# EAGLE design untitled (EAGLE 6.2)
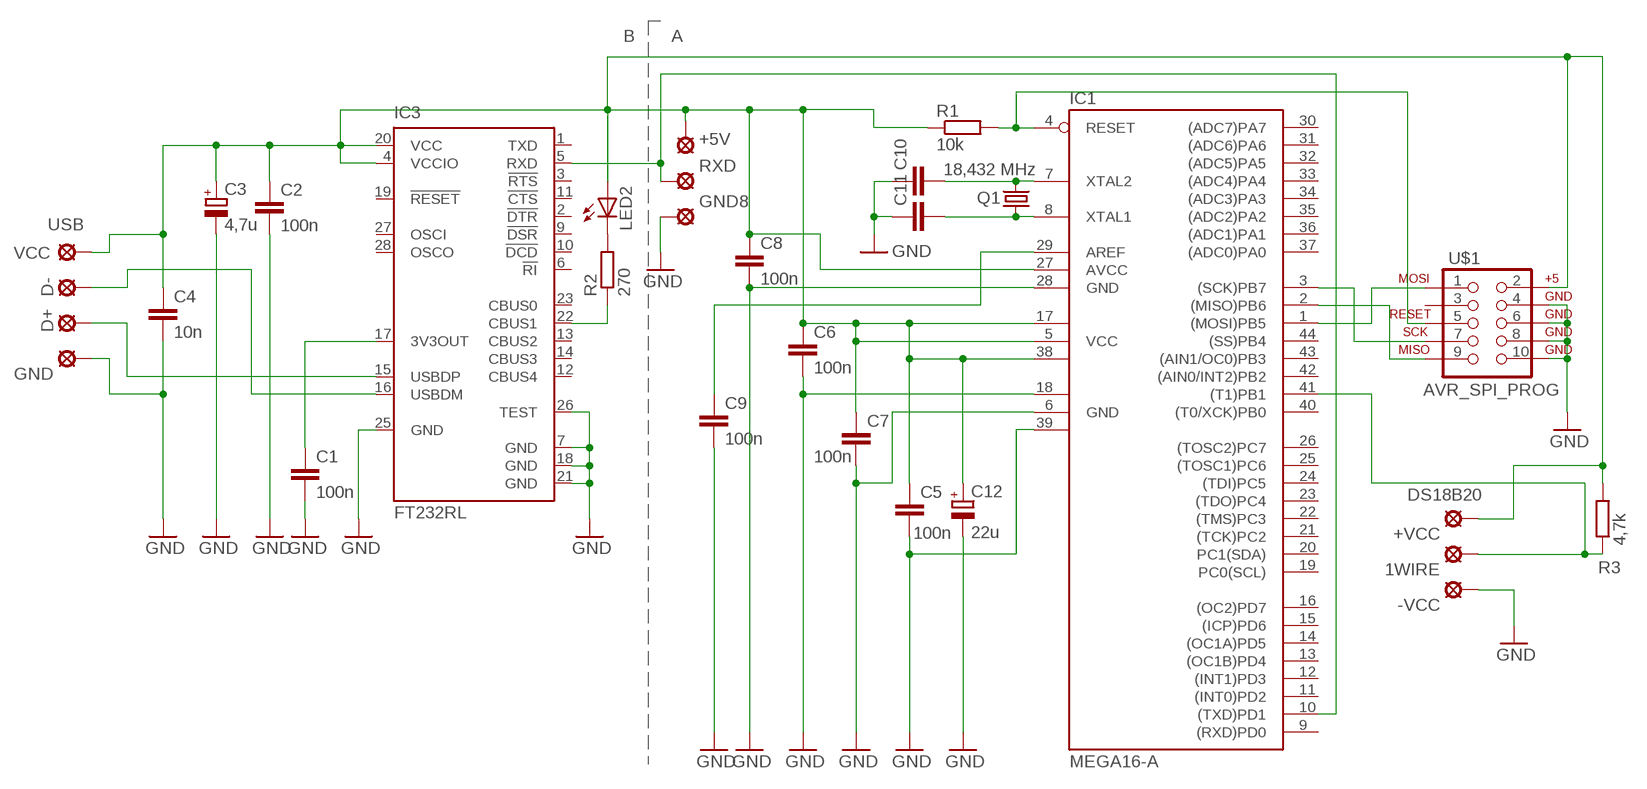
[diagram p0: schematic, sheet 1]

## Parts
1WIRE  LSP11  [LSP11]
+5V  LSP11  [LSP11]
+VCC  LSP11  [LSP11]
-VCC  LSP11  [LSP11]
C1  100n  C-EUC1210  [C1210]
C2  100n  C-EUC1210  [C1210]
C3  4,7u  CPOL-EU153CLV-0405  [153CLV-0405]
C4  10n  C-EUC1206  [C1206]
C5  100n  C-EUC1210  [C1210]
C6  100n  C-EUC1210  [C1210]
C7  100n  C-EUC1210  [C1210]
C8  100n  C-EUC1210  [C1210]
C9  100n  C-EUC1210  [C1210]
C10  C-EUC1206  [C1206]
C11  C-EUC1206  [C1206]
C12  22u  CPOL-EUUD-6,3X7,7  [UD-6,3X7,7_NICHICON]
D+  LSP11  [LSP11]
D-  LSP11  [LSP11]
GND  LSP11  [LSP11]
GND8  LSP11  [LSP11]
IC1  MEGA16-A  [TQFP44]
IC3  FT232RL  [SSOP28]
LED2  LED-FKIT-1206  [FKIT-LED-1206]
Q1  18,432 MHz  CRYSTALHC49S  [HC49/S]
R1  10k  R-EU_R1206  [R1206]
R2  270  R-EU_R1206  [R1206]
R3  4,7k  R-EU_R1206  [R1206]
RXD  LSP11  [LSP11]
U$1  AVR_SPI_PROG  [AVR_ICSP]
VCC  LSP11  [LSP11]

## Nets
GND: -VCC.MP C1.2 C2.2 C3.- C4.2 C5.2 C6.2 C7.2 C8.2 C9.2 C10.1 C11.1 C12.- GND8.MP GND.MP IC1.6(GND) IC1.18(GND1) IC1.28(GND) IC1.39(GND2) IC3.7(GND) IC3.18(GND) IC3.21(GND) IC3.25(GND) IC3.26(TEST) U$1.4 U$1.6 U$1.8 U$1.10
N$1: C1.1 IC3.17(3V3OUT)
N$2: D-.MP IC3.16(USBDM)
N$3: +5V.MP +VCC.MP C2.1 C3.+ C4.1 C5.1 C6.1 C7.1 C8.1 C12.+ IC1.5(VCC) IC1.17(VCC1) IC1.27(AVCC) IC1.38(VCC2) IC3.4(VCCIO) IC3.20(VCC) LED2.A R1.1 R3.2 U$1.2 VCC.MP
N$4: IC1.10((TXD)PD1) IC3.5(RXD) RXD.MP
N$5: IC1.1((MOSI)PB5) U$1.1
N$6: D+.MP IC3.15(USBDP)
N$7: IC1.3((SCK)PB7) U$1.7
N$8: IC3.22(CBUS1) R2.1
N$9: C10.2 IC1.7(XTAL2) Q1.2
N$10: LED2.C R2.2
N$11: C11.2 IC1.8(XTAL1) Q1.1
N$12: IC1.4(RESET) R1.2 U$1.5
N$13: IC1.2((MISO)PB6) U$1.9
N$14: C9.1 IC1.29(AREF)
N$16: 1WIRE.MP IC1.41((T1)PB1) R3.1
Unconnected: IC1.9((RXD)PD0) IC1.11((INT0)PD2) IC1.12((INT1)PD3) IC1.13((OC1B)PD4) IC1.14((OC1A)PD5) IC1.15((ICP)PD6) IC1.16((OC2)PD7) IC1.19(PC0(SCL)) IC1.20(PC1(SDA)) IC1.21((TCK)PC2) IC1.22((TMS)PC3) IC1.23((TDO)PC4) IC1.24((TDI)PC5) IC1.25((TOSC1)PC6) IC1.26((TOSC2)PC7) IC1.30((ADC7)PA7) IC1.31((ADC6)PA6) IC1.32((ADC5)PA5) IC1.33((ADC4)PA4) IC1.34((ADC3)PA3) IC1.35((ADC2)PA2) IC1.36((ADC1)PA1) IC1.37((ADC0)PA0) IC1.40((T0/XCK)PB0) IC1.42((AIN0/INT2)PB2) IC1.43((AIN1/OC0)PB3) IC1.44((SS)PB4) IC3.1(TXD) IC3.2(!DTR) IC3.3(!RTS) IC3.6(!RI) IC3.9(!DSR) IC3.10(!DCD) IC3.11(!CTS) IC3.12(CBUS4) IC3.13(CBUS2) IC3.14(CBUS3) IC3.19(!RESET) IC3.23(CBUS0) IC3.27(OSCI) IC3.28(OSCO) U$1.3

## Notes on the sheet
- B | A
- USB
- DS18B20

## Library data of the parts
1WIRE +5V +VCC -VCC D+ D- GND GND8 RXD VCC = solpad:LSP11: SOLDER PAD
C1 C2 C4-C11 = rcl:C-EU: CAPACITOR, European symbol
C3 C12 = rcl:CPOL-EU: POLARIZED CAPACITOR, European symbol
IC1 = atmel:MEGA16: MICROCONTROLLER 16 Kbytes FLASH 1 kbytes SRAM 512 bytes EEPROM USART 8-channel 10 bit ADC Source: avr.lbr; MPN: ATMEGA16-16AU; OC_FARNELL: 9171134; OC_NEWARK: 96K6515
IC3 = ftdichip:FT232R: Source: http://www.ftdichip.com/Documents/DataSheets/DS_FT232R_v104.pdf; MPN: FT232RL; OC_FARNELL: 1146032; OC_NEWARK: 91K9918
LED2 = SparkFun:LED: LEDs
Q1 = crystal:CRYSTAL: CRYSTAL; OC_FARNELL: 1667008; OC_NEWARK: unknown
R1-R3 = rcl:R-EU_: RESISTOR, European symbol
U$1 = SparkFun:AVR_SPI_PROG: AVR ICSP Header This is the standard AVR In Circuit Serial Programming header. Minimal, but includes pin one indicator. Works with standard Olimex programmers. Also look for the 6-pin reduced version. Spark Fun Electronics SKU: PRT-00778

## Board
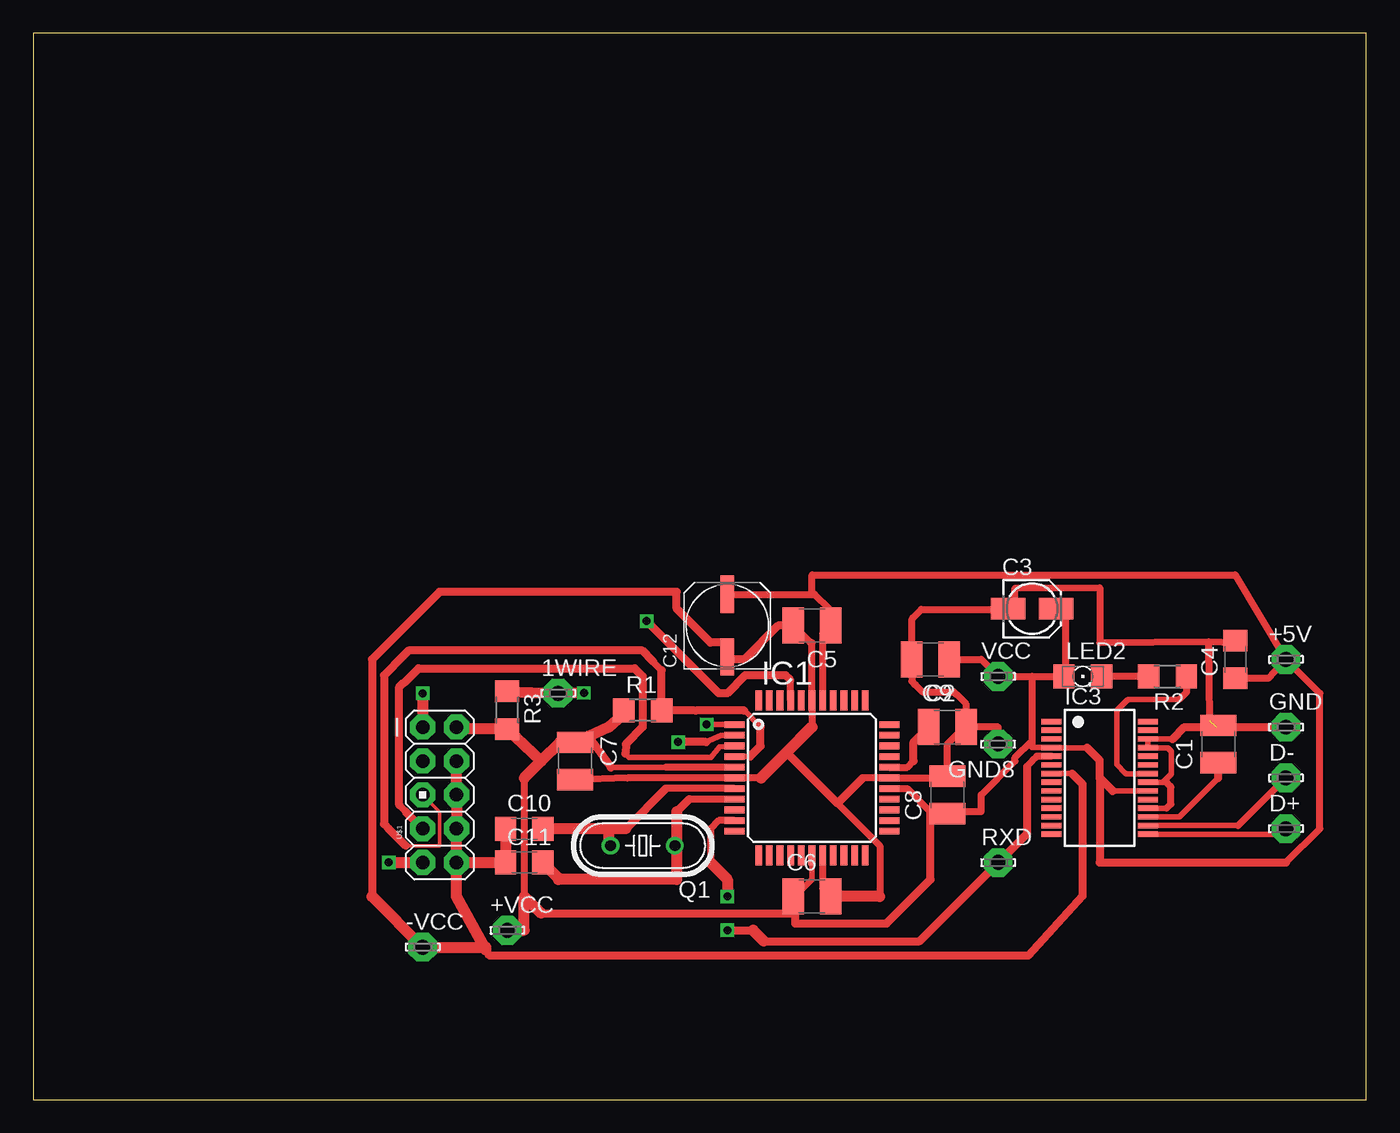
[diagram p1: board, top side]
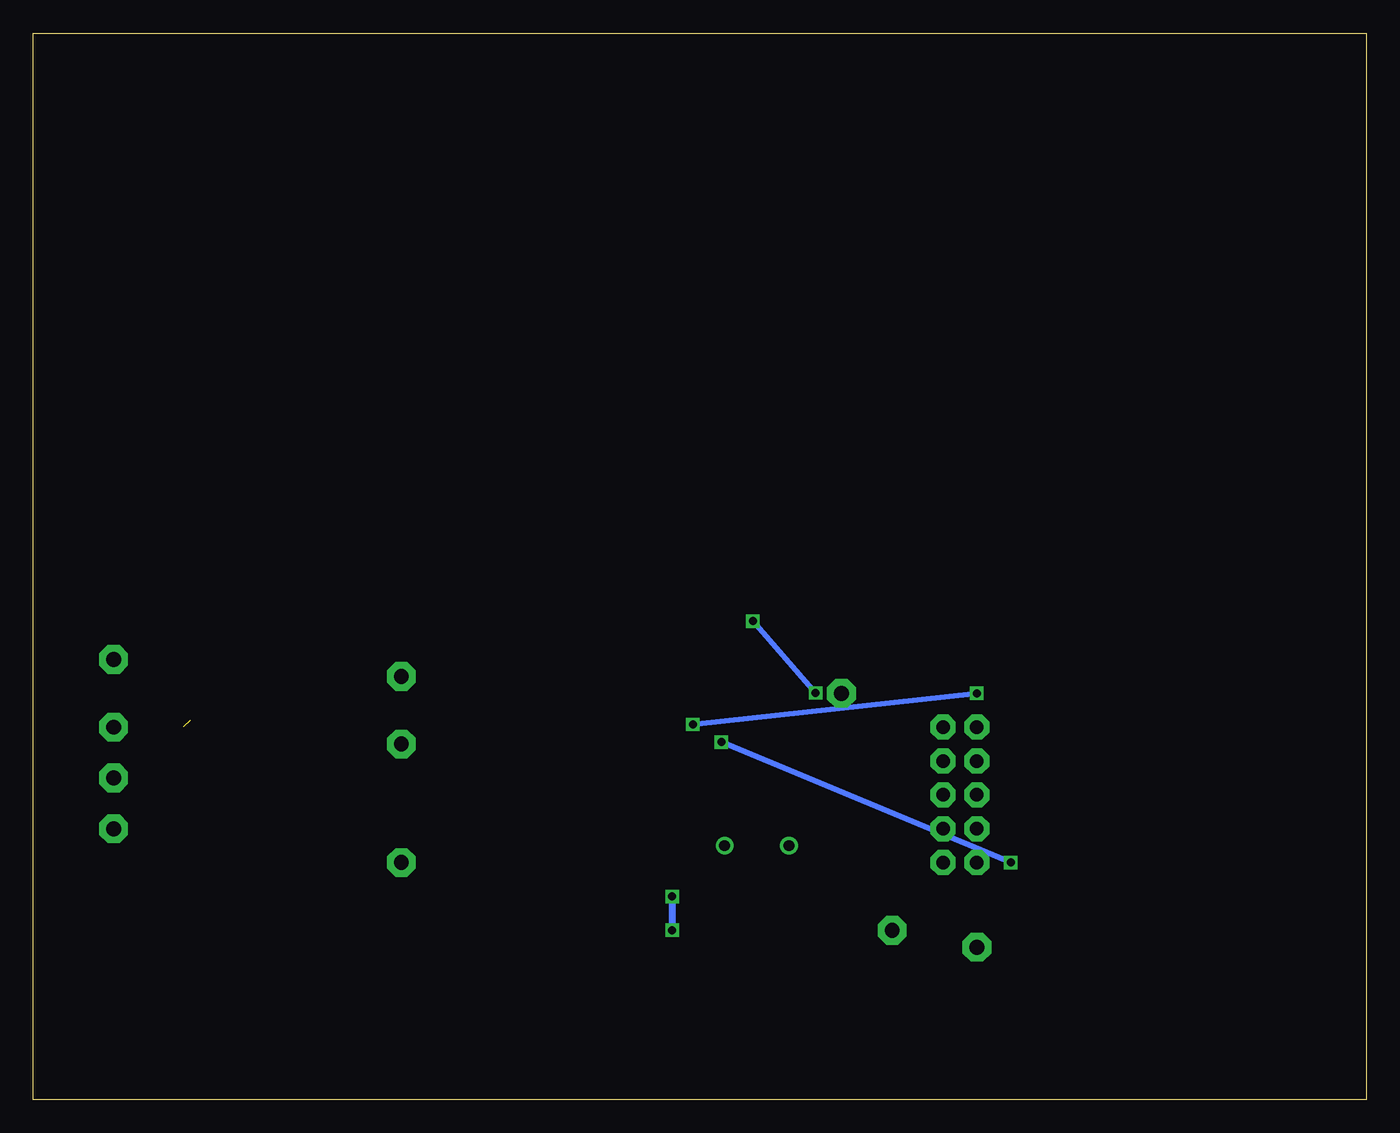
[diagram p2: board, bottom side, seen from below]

Size 100 x 80 mm. Coordinates in mm from the lower left corner, seen from the top.
Outline: 0,0 100,0 100,80 0,80 0,0
Copper layers (1*16): Top 0.035mm / dielectric 1.5mm / Bottom 0.035mm
Design rules: minimum track width 10mil, minimum drill 24mil, track to track 8mil, track to pad 8mil, pad to pad 8mil, via to via 8mil, smd to smd 8mil, copper to edge 40mil, drill to drill 8mil, minimum pad ring 10mil, minimum via ring 8mil, stop-mask expansion 4mil, vias tented up to drill 0mil, thermal gap 10mil

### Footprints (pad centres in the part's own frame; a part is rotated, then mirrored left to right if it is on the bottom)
LSP11 = drill 1.118 pad 2.159 octagon: MP 0,0
C1210 = smd 1.6 x 2.7: 1 -1.4,0; 2 1.4,0
153CLV-0405 = smd 2.6 x 1.6: + 1.8,0; - -1.8,0
C1206 = smd 1.6 x 1.8: 1 -1.4,0; 2 1.4,0
UD-6,3X7,7_NICHICON = smd 2.8 x 1: + 2.35,0; - -2.35,0
TQFP44 = smd 1.5 x 0.5: 1 -5.8,4; 2 -5.8,3.2; 3 -5.8,2.4; 4 -5.8,1.6; 5 -5.8,0.8; 6 -5.8,0; 7 -5.8,-0.8; 8 -5.8,-1.6; 9 -5.8,-2.4; 10 -5.8,-3.2; 11 -5.8,-4; 23 5.8,-4; 24 5.8,-3.2; 25 5.8,-2.4; 26 5.8,-1.6; 27 5.8,-0.8; 28 5.8,0; 29 5.8,0.8; 30 5.8,1.6; 31 5.8,2.4; 32 5.8,3.2; 33 5.8,4 | smd 0.5 x 1.5: 12 -4,-5.8; 13 -3.2,-5.8; 14 -2.4,-5.8; 15 -1.6,-5.8; 16 -0.8,-5.8; 17 0,-5.8; 18 0.8,-5.8; 19 1.6,-5.8; 20 2.4,-5.8; 21 3.2,-5.8; 22 4,-5.8; 34 4,5.8; 35 3.2,5.8; 36 2.4,5.8; 37 1.6,5.8; 38 0.8,5.8; 39 0,5.8; 40 -0.8,5.8; 41 -1.6,5.8; 42 -2.4,5.8; 43 -3.2,5.8; 44 -4,5.8
SSOP28 = smd 0.4 x 1.5: 1 -4.225,-3.625; 2 -3.575,-3.625; 3 -2.925,-3.625; 4 -2.275,-3.625; 5 -1.625,-3.625; 6 -0.975,-3.625; 7 -0.325,-3.625; 8 0.325,-3.625; 9 0.975,-3.625; 10 1.625,-3.625; 11 2.275,-3.625; 12 2.925,-3.625; 13 3.575,-3.625; 14 4.225,-3.625; 15 4.225,3.625; 16 3.575,3.625; 17 2.925,3.625; 18 2.275,3.625; 19 1.625,3.625; 20 0.975,3.625; 21 0.325,3.625; 22 -0.325,3.625; 23 -0.975,3.625; 24 -1.625,3.625; 25 -2.275,3.625; 26 -2.925,3.625; 27 -3.575,3.625; 28 -4.225,3.625
FKIT-LED-1206 = smd 1.6 x 1.803: A -1.422,0; C 1.422,0
HC49/S = drill 0.813: 1 -2.413,0; 2 2.413,0
R1206 = smd 1.6 x 1.803: 1 -1.422,0; 2 1.422,0
AVR_ICSP = drill 1.016 pad 1.88 octagon: 1 -1.27,5.08; 2 1.27,5.08; 3 -1.27,2.54; 4 1.27,2.54; 5 -1.27,0; 6 1.27,0; 7 -1.27,-2.54; 8 1.27,-2.54; 9 -1.27,-5.08; 10 1.27,-5.08

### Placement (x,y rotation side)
1WIRE  39.37,30.48 0 top
+5V  93.98,33.02 0 top
+VCC  35.56,12.7 0 top
-VCC  29.21,11.43 0 top
C1  88.9,26.67 90 top
C2  67.31,33.02 180 top
C3  74.93,36.83 0 top
C4  90.17,33.02 90 top
C5  58.42,35.56 180 top
C6  58.42,15.24 0 top
C7  40.64,25.4 270 top
C8  68.58,22.86 90 top
C9  68.58,27.94 0 top
C10  36.83,20.32 0 top
C11  36.83,17.78 0 top
C12  52.07,35.56 90 top
D+  93.98,20.32 0 top
D-  93.98,24.13 0 top
GND  93.98,27.94 0 top
GND8  72.39,26.67 180 top
IC1  58.42,24.13 0 top
IC3  80.01,24.13 270 top
LED2  78.74,31.75 0 top
Q1  45.72,19.05 180 top
R1  45.72,29.21 0 top
R2  85.09,31.75 180 top
R3  35.56,29.21 270 top
RXD  72.39,17.78 0 top
U$1  30.48,22.86 0 top
VCC  72.39,31.75 0 top

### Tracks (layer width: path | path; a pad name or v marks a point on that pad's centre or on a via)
GND  (1 unrouted)
  Top 0.254: 35.56,17.78 C11.1 | 35.56,20.32 C10.1 | 90.17,34.29 C4.2 | 67.31,36.83 C3.- 73.66,36.83 | 53.34,24.13 IC1.6 | 58.42,29.21 IC1.39 | 59.69,15.24 C6.2 | 63.5,24.13 IC1.28 | 69.85,27.94 C9.2 | 68.58,24.13 C8.2 | 52.07,34.29 C12.- | 88.9,27.94 C1.2
  Top 0.406: IC3.18 85.03,21.86 | 85.09,23.72 85.01,23.8 IC3.21 84.74,23.8 85.37,24.43 85.37,26.11 85.11,26.36 83.67,26.36 IC3.25 IC3.26 85.47,27.05 | 88.77,27.94 C1.2 | IC3.7 77.93,24.45 | 33.96,11.43 33.96,11.21
  Top 0.508: IC1.39 58.42,34.29 58.29,34.29 C5.2 | 52.26,33.02 C12.- | IC1.28 68.45,24.13 C8.2 68.58,26.67 69.85,27.94 | 88.16,34.37 90.17,34.29 | GND8.MP 72.39,27.94 C9.2 69.95,27.97 69.95,29.72 69.24,30.43 69.22,30.43 69.06,30.58 66.7,30.58 66.19,31.09 66.19,31.11 65.91,31.4 C2.2 65.91,36.01 65.99,36.09 65.99,36.14 66.62,36.78 73.08,36.78 C3.- | 63.5,15.24 63.5,19.05 60.33,22.23 | 88.16,34.37 80.01,34.29 80.01,38.41 73.66,38.38 73.66,36.83 | 85.03,21.86 85.34,22.17 85.34,23.44 85.32,23.47 85.32,23.5 85.09,23.72 | 63.5,24.13 62.23,24.13 | 58.42,29.21 58.42,27.94 58.4,27.94 | 54.61,24.13 53.34,24.13 | 56.49,26.04 56.52,26.04 | IC1.18 59.22,15.84 C6.2 | IC1.6 44.58,24.13 C7.2 | 88.16,34.37 88.24,28.45
  Top 0.61: C5.2 55.88,35.56 53.34,33.02 52.26,33.02 | 88.9,27.94 GND.MP | 85.47,27.05 86.36,27.94 88.77,27.94 | 62.23,24.13 60.33,22.23 56.52,26.04 | 77.93,24.45 78.72,23.67 78.72,15.27 74.62,10.79 34.24,10.79 33.96,11.21 | 52.07,34.29 50.8,34.29 48.26,36.83 48.26,38.1 30.48,38.1 25.4,33.02 25.4,15.24
  Top 0.813: C10.1 C11.1 U$1.10 | U$1.4 U$1.6 U$1.8 U$1.10 | 63.5,15.24 C6.2 | U$1.10 31.75,15.24 33.96,11.21 | 58.42,27.94 54.61,24.13 | 58.4,27.94 56.49,26.04 | 33.96,11.43 -VCC.MP 25.4,15.24
N$1
  Top 0.406: IC3.17 85.97,21.2 88.9,24.13
  Top 0.61: 88.9,24.13 C1.1
N$2
  Top 0.406: IC3.16 90.41,20.55
  Top 0.508: 90.41,20.55 D-.MP
N$3
  Top 0.254: 77.47,36.83 C3.+ | 77.47,31.75 LED2.A | 68.58,21.59 C8.1 67.31,21.59 | 57.15,15.24 C6.1
  Top 0.406: IC1.17 58.42,16.51 57.15,15.24 | IC3.20 80.98,23.16 | 79.07,26.39 IC3.4 74.93,26.41 74.93,26.67 | 47.46,24.93 43.33,24.92
  Top 0.508: IC1.38 59.23,29.93 59.23,34.97 C5.1 59.69,35.69 59.69,36.83 58.61,37.91 58.42,37.91 | C12.+ 58.42,37.91 | IC1.27 65.57,23.33 67.31,21.59 68.45,21.59 C8.1 | +5V.MP 90.17,39.37 58.42,39.37 58.42,37.91 | 74.93,31.75 VCC.MP 71.12,33.02 C2.1 | 74.93,31.75 LED2.A | 77.47,31.75 77.47,36.83 | 68.58,21.59 71.12,21.59 71.12,22.86 73.66,25.4 73.66,25.65 74.93,26.92 | 74.93,31.75 74.93,26.92 | 74.93,26.92 74.93,26.67 | 57.15,15.24 57.15,13.97 | +5V.MP 96.52,30.48 96.52,20.32 93.98,17.78 | 39.5,26.8 C7.1 41.65,27.25 | 36.83,24.13 36.83,15.24 | R1.1 44.15,28.78 | IC1.5 47.46,24.93 | C4.1 92.69,31.62 +5V.MP
  Top 0.61: 80.98,23.16 80.01,24.13 | 80.01,24.13 80.01,25.45 79.07,26.39 | 93.98,17.78 80.01,17.78 80.01,24.13 | 38.1,13.97 57.15,13.97 57.15,13.21 64.01,13.21 67.31,16.51 67.31,21.59 | 43.33,24.92 41.65,27.25
  Top 0.813: 39.5,26.8 38.1,25.4 | 38.1,25.4 36.83,24.13 | 38.1,13.97 36.83,15.24 36.83,12.7 +VCC.MP | 44.15,28.78 43.18,27.94 41.65,27.25 | 38.1,25.4 R3.2 31.9,27.79 U$1.2
N$4  (via drill 0.6)
  Top 0.508: IC3.5 75.28,25.75 74.93,25.4 74.93,25.38 74.55,24.99 | IC1.10 51.41,20.93 50.8,20.32 50.8,17.78
  Top 0.61: 74.55,24.99 74.55,19.94 RXD.MP 66.5,11.89 54.81,11.89 | v52.07,12.7 54,12.7
  Top 0.813: 50.8,17.78 52.07,16.51 v52.07,15.24 | 54,12.7 54.81,11.89
  Bottom 0.508: v52.07,15.24 v52.07,12.7
N$5  (via drill 0.6)
  Top 0.406: IC1.1 v50.52,28.14
  Top 0.813: v29.21,30.48 U$1.1
  Bottom 0.406: v50.52,28.14 v29.21,30.48
N$6
  Top 0.406: IC3.15 93.56,19.91 D+.MP
N$7
  Top 0.254: 52.07,26.67 IC1.3
  Top 0.406: 44.42,25.96 44.7,25.65 50.85,25.68 51.49,26.44 IC1.3
  Top 0.508: 27.94,21.59 27.94,21.61 27.46,22.1 | 27.79,31.29 27.84,31.29
  Top 0.61: U$1.7 27.94,21.59 | 44.42,25.96 44.45,26.67 45.72,27.94 45.72,31.75 45.11,32.36 28.91,32.36 27.84,31.29 | 27.46,22.1 27.46,30.96 27.79,31.29
N$8
  Top 0.406: 85.98,30.02 82.17,30.02 82.14,30 82.07,30 81.28,29.21 81.28,25.15 81.94,24.49 81.97,24.49 82.02,24.43 83.61,24.43 IC3.22
  Top 0.508: R2.1 86.51,30.56 85.98,30.02
N$9
  Top 0.254: 38.1,20.32 C10.2 | 43.18,19.05 Q1.2
  Top 0.508: IC1.7 47.46,23.33
  Top 0.61: 47.46,23.33 44.45,20.32
  Top 0.813: 43.18,20.32 C10.2 | 43.18,19.05 43.18,20.32 | 44.45,20.32 43.18,20.32
N$10
  Top 0.254: 80.01,31.75 LED2.C | 83.82,31.75 R2.2
  Top 0.508: R2.2 LED2.C
N$11
  Top 0.254: 38.1,17.78 C11.2 | 48.26,19.05 Q1.1
  Top 0.508: IC1.8 49.2,22.53 | 48.26,19.18 Q1.1
  Top 0.61: 49.2,22.53 48.26,21.59 | 39.37,16.51 39.37,16.64
  Top 0.813: 48.26,19.05 48.26,16.51 39.37,16.51 | 48.26,21.59 48.26,19.18 | 39.37,16.64 C11.2
N$12
  Top 0.254: 27.94,19.05 30.48,19.05 30.48,21.59 U$1.5
  Top 0.406: IC1.4 53.77,25.73 | 54.56,27.96 53.34,29.18 | 49.71,29.18 R1.2
  Top 0.508: 47.14,32.21 46.51,32.84 46.51,32.87 | 27.76,33.3 27.76,33.27
  Top 0.61: 27.94,19.05 26.67,20.32 26.31,20.68 26.31,31.83 27.76,33.27 | 49.53,29.21 R1.2 47.14,32.21 | 53.77,25.73 54.56,26.52 54.56,27.96 | 53.34,29.18 49.71,29.18 | 46.51,32.87 45.7,33.68 28.14,33.68 27.76,33.3
N$13  (via drill 0.6)
  Top 0.406: IC1.2 51.59,27.33 50.47,26.82
  Top 0.61: 50.47,26.82 v48.39,26.82
  Top 0.813: v26.67,17.78 U$1.9
  Bottom 0.406: v48.39,26.82 v26.67,17.78
N$14
  Top 0.508: IC1.29 65.57,24.93 66.04,25.4
  Top 0.61: 66.04,25.4 66.04,26.8 C9.1
N$16  (via drill 0.6)
  Top 0.406: 51.46,30.48 51.44,30.5 51.41,30.5 | 56.82,31.47 56.79,31.47 | 53.42,31.83 53.37,31.77 | IC1.41
  Top 0.508: IC1.41 56.82,31.47
  Top 0.61: 53.37,31.77 52.07,30.48 51.46,30.48 | 51.41,30.5 v46.02,35.89 | 56.79,31.47 56.44,31.83 53.42,31.83
  Top 0.813: v41.3,30.5 1WIRE.MP R3.1
  Bottom 0.406: v46.02,35.89 v41.3,30.5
